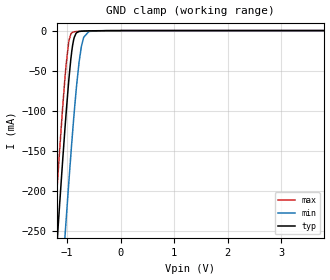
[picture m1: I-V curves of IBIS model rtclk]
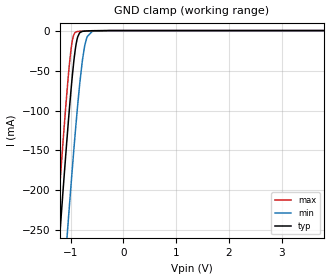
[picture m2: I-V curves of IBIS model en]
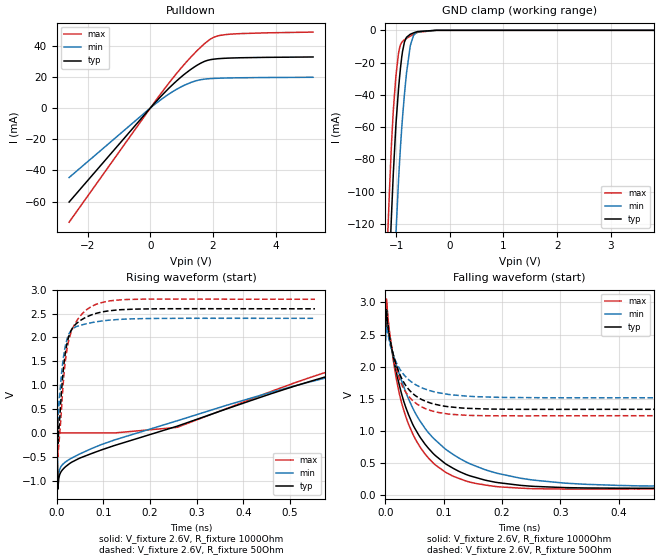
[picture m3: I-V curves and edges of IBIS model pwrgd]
|Texas Instruments Incorporated
| automotive Catalog 2.95V to 6V Input, 4A, 2MHz Synchronous Step Down
| SWIFT(tm) DCDC Converter
| Marketing part#   Digital Voltage Range   Package-type   #pins
| TPS57114QRTERQ1   2.95V-6V   QFN   16
[IBIS Ver]   4.1
[File name]   tps57114.ibs
[File Rev]   1.1
[Date]   8/06/2014
[Source]
| Texas Instruments Incorporated.
| Analog-eLab Design Center, HPA
| 12500 TI Blvd
| Dallas, TX -75243
[Notes]   Revision History:
| Rev 1.1: 8/06/2014
| - Added en, pwrgd models.
| Rev 1.0: 7/30/2014
| - Initial version of the model
| - Model generated from simulations in TISPICE
| - Model matched to SPICE simulation
| - C_comp although listed in numerical order of value are
|   obtained from varying PVT conditions. For PVT conditions for
|   each specific value refer the buffer description under
|   respective [Model]. IBIS model user is responsible for using
|   appropriate C_comp to simulate for Signal Integrity.
[Disclaimer]
| This model is designed as an aid for customers of Texas Instruments.
| TI and its licensors and suppliers make no warranties, either expressed
| or implied, with respect to this  model, including the warranties of
| merchantability or fitness for a particular purpose. The model is
| provided solely on an "as is" basis. The entire risk as to its quality
| and performance is with the customer.
[Copyright]
(C) Copyright 2014 Texas Instruments Incorporated.All rights reserved.
|   TPS57114
[Component]   TPS57114RTE
[Manufacturer]   TI
[Package]   |16 QFN  -  RTE package
|   typ   min   max
R_pkg   0.02609   0.02582   0.02655
L_pkg   0.81078nH   0.79906nH   0.82662nH
C_pkg   0.15670pF   0.14661pF   0.16188pF
[Pin]  signal_name   model_name   R_pin   L_pin   C_pin
1   VIN   power   0.01187   0.75296nH  0.26060pF
2   VIN   power   0.01171   0.71361nH  0.26727pF
3   GND   gnd   0.01169   0.71205nH  0.26671pF
4   GND   gnd   0.01220   0.73983nH  0.28477pF
5   GND   gnd   0.03032   0.96192nH  0.16334pF
6   VSENSE   nc   0.02662   0.83091nH  0.16437pF
7   COMP   nc   0.02547   0.78920nH  0.15897pF
8   RT/CLK   rtclk   0.02655   0.82662nH  0.14661pF
9   SS/TR   nc   0.02579   0.79643nH  0.14300pF
10   PH   nc   0.01088   0.65997nH  0.25329pF
11   PH   nc   0.01090   0.63864nH  0.27183pF
12   PH   nc   0.01125   0.71480nH  0.24611pF
13   BOOT   nc   0.02895   0.90385nH  0.15593pF
14   PWRGD   pwrgd   0.02582   0.79906nH  0.16162pF
15   EN   en   0.02591   0.80666nH  0.16188pF
16   VIN   power   0.02908   0.91969nH  0.15877pF
| Models and submodels in the file (3): rtclk (Input), en (Input), pwrgd (Open_drain)
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|   rtclk Model
[Model]   rtclk
Model_type   Input
Vinl = 0.4
Vinh = 2.5
|   typ   min   max
|   (nom PVT)   (fast PVT)   (slow PVT)
C_comp   1.701e-13   1.679e-13   1.709e-13
| Where nom  PVT is Nominal Process, 2.6V, 27C
|   Fast PVT is Strong Process,  2.8V, -40C
|   Slow PVT is Weak Process,   2.4V, 150C
[Voltage Range]   2.6   2.4   2.8
|Junction Temperature
[Temperature Range]   27   150   -40
[Power Clamp Reference]   2.6   2.4   2.8
[GND Clamp Reference]   0   0   0
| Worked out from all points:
|   GND clamp passes 1 mA (typ) near -0.77 V on its own axis
[GND Clamp]
|   Voltage   I(typ)   I(min)   I(max)
-2.6V     -1.785A    -1.914A    -1.724A
-1.269V   -345mA     -484.1mA   -276.9mA
-1.232V   -307.3mA   -446.4mA   -239.1mA
-1.169V   -243.8mA   -382.6mA   -175.9mA
-1.045V   -124.9mA   -260mA     -61.44mA
-1.024V   -105.6mA   -239.3mA   -44.69mA
-972.8mV  -63.71mA   -191.7mA   -14.71mA
-898.4mV  -18.16mA   -125.9mA   -2.023mA
-826.4mV  -2.757mA   -69.8mA    -1.176mA
-735.2mV  -741uA     -19.94mA   -820.7uA
-593.6mV  -320.7uA   -1.006mA   -410.6uA
5.2V      0A         0A         0A
[POWER Clamp]
|   Voltage   I(typ)   I(min)   I(max)
-2.6V     0A         0A         0A
0V        0A         0A         0A
5.2V      0A         0A         0A
|   en Model
[Model]   en
Model_type   Input
Vinl = 0.4
Vinh = 2.5
|   typ   min   max
|   (nom PVT)   (fast PVT)   (slow PVT)
C_comp   1.654e-13   1.644e-13   1.679e-13
| Where nom  PVT is Nominal Process, 2.6V, 27C
|   Fast PVT is Strong Process,  2.8V, -40C
|   Slow PVT is Weak Process,   2.4V, 150C
[Voltage Range]   2.6   2.4   2.8
|Junction Temperature
[Temperature Range]   27   150   -40
[Power Clamp Reference]   2.6   2.4   2.8
[GND Clamp Reference]   0   0   0
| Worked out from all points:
|   GND clamp passes 1 mA (typ) near -0.78 V on its own axis
[GND Clamp]
|   Voltage   I(typ)   I(min)   I(max)
-2.6V     -1.608A    -1.726A    -1.554A
-1.266V   -310.5mA   -436.6mA   -248.7mA
-1.232V   -278.9mA   -405.1mA   -217.1mA
-1.172V   -224.3mA   -350.2mA   -162.6mA
-1.085V   -148mA     -272.3mA   -87.92mA
-1.043V   -112.4mA   -235mA     -54.82mA
-970.4mV  -57.53mA   -173.6mA   -12.98mA
-897mV    -16.81mA   -115.1mA   -1.668mA
-824mV    -2.466mA   -63.66mA   -865uA
-732.8mV  -615.5uA   -18.38mA   -530.6uA
-591.2mV  -215.8uA   -921.1uA   -150.8uA
5.2V      0A         0A         0A
[POWER Clamp]
|   Voltage   I(typ)   I(min)   I(max)
-2.6V     0A         0A         0A
0V        0A         0A         0A
5.2V      0A         0A         0A
|   pwrgd Model
[Model]   pwrgd
Model_type   Open_drain
Polarity   Inverting
Vmeas = 1.3
Vref = 2.6
Cref = 2pF
Rref = 100
|   typ   min   max
|   (nom PVT)   (fast PVT)   (slow PVT)
C_comp   3.259e-13   2.888e-13   3.619e-13
| Where nom  PVT is Nominal Process, 2.6V, 27C
|   Fast PVT is Strong Process,  2.8V, -40C
|   Slow PVT is Weak Process,   2.4V, 150C
[Voltage Range]   2.6   2.4   2.8
|Junction Temperature
[Temperature Range]   27   125   -40
[Pullup Reference]   2.6   2.4   2.8
[Pulldown Reference]   0   0   0
[Power Clamp Reference]   2.6   2.4   2.8
[GND Clamp Reference]   0   0   0
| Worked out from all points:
|   slope of the pulldown table from 0 to 0.39 V, typ, clamps not added: 45.7 ohm
|   GND clamp passes 1 mA (typ) near -0.62 V on its own axis
|   falling waveform, V_fixture 2.6V, R_fixture 1000Ohm: 20-80 % time 71.7ps typ, 102ps min, 56.8ps max; typ from 2.6 V to 0.11 V
|   rising waveform, V_fixture 2.6V, R_fixture 1000Ohm: 20-80 % time 651ps typ, 685ps min, 624ps max; typ from 0.11 V to 2.6 V
|   falling waveform, V_fixture 2.6V, R_fixture 50Ohm: 20-80 % time 36.6ps typ, 45.5ps min, 31.3ps max; typ from 2.6 V to 1.33 V
|   rising waveform, V_fixture 2.6V, R_fixture 50Ohm: 20-80 % time 32.4ps typ, 25.3ps min, 34.7ps max; typ from 1.33 V to 2.6 V
[Pulldown]
|   Voltage   I(typ)   I(min)   I(max)
-2.6V     -60.31mA   -44.62mA   -73.23mA
0V        0A         0A         0A
362.4mV   7.97mA     5.688mA    9.925mA
755.2mV   15.79mA    10.96mA    20.06mA
1.11V     21.95mA    14.76mA    28.54mA
1.51V     27.57mA    17.67mA    37.06mA
1.832V    30.51mA    18.65mA    42.83mA
2.121V    31.46mA    18.99mA    45.96mA
2.546V    31.96mA    19.22mA    47.25mA
5.2V      32.64mA    19.64mA    48.59mA
[GND Clamp]
|   Voltage   I(typ)   I(min)   I(max)
-2.6V     -1.679A    -1.742A    -1.651A
-1.15V    -168.7mA   -250.5mA   -120.9mA
-1.091V   -118mA     -197.7mA   -73.51mA
-1.052V   -88.15mA   -164.2mA   -49.32mA
-1.001V   -57.14mA   -124.5mA   -27.39mA
-941.6mV  -31.06mA   -84.74mA   -11.68mA
-881.4mV  -13.22mA   -54.21mA   -6.899mA
-807.2mV  -4.322mA   -26.62mA   -4.999mA
-735.8mV  -2.419mA   -9.464mA   -3.555mA
-624.8mV  -1.007mA   -1.336mA   -1.624mA
-260mV    -246.8nA   -3.093uA   -51.13nA
5.2V      0A         0A         0A
[POWER Clamp]
|   Voltage   I(typ)   I(min)   I(max)
-2.6V     0A         0A         0A
0V        0A         0A         0A
5.2V      0A         0A         0A
[Ramp]
R_load = 1000
|   typ   min   max
dV/dt_r   1.49325/6.49618e-10   1.35616/6.82854e-10   1.62132/6.2478e-10
dV/dt_f   1.4939/7.16963e-11   1.35674/1.01541e-10   1.6218/5.68186e-11
[Falling Waveform]
V_fixture = 2.6V
V_fixture_min = 2.4V
V_fixture_max = 2.8V
R_fixture = 1000Ohm
|   Time   V(typ)   V(min)   V(max)
0s        2.6V       2.4V       2.8V
2ps       2.899V     2.732V     3.053V
8ps       2.429V     2.387V     2.468V
20ps      1.863V     1.989V     1.749V
34ps      1.388V     1.624V     1.248V
50ps      1.044V     1.297V     893.4mV
86ps      610mV      852.4mV    464.2mV
146ps     293.5mV    480.5mV    196mV
344ps     107.3mV    164.4mV    88.81mV
1.096ns   110.3mV    138.2mV    97.27mV
[Rising Waveform]
V_fixture = 2.6V
V_fixture_min = 2.4V
V_fixture_max = 2.8V
R_fixture = 1000Ohm
|   Time   V(typ)   V(min)   V(max)
0s        110.1mV    138.7mV    96.97mV
2ps       -1.178V    -1.054V    0V
8ps       -827.8mV   -716.7mV   0V
32ps      -611.5mV   -524.6mV   0V
258ps     140.6mV    254.1mV    117mV
624ps     1.305V     1.26V      1.413V
914ps     1.918V     1.781V     2.093V
1.32ns    2.349V     2.16V      2.553V
2.042ns   2.56V      2.358V     2.763V
3.998ns   2.599V     2.399V     2.799V
[Falling Waveform]
V_fixture = 2.6V
V_fixture_min = 2.4V
V_fixture_max = 2.8V
R_fixture = 50Ohm
|   Time   V(typ)   V(min)   V(max)
0s        2.6V       2.4V       2.8V
2ps       2.861V     2.692V     3.02V
6ps       2.519V     2.427V     2.605V
12ps      2.241V     2.216V     2.248V
20ps      1.989V     2.039V     1.925V
30ps      1.779V     1.893V     1.68V
50ps      1.557V     1.728V     1.445V
78ps      1.43V      1.621V     1.314V
190ps     1.337V     1.522V     1.232V
554ps     1.335V     1.515V     1.235V
[Rising Waveform]
V_fixture = 2.6V
V_fixture_min = 2.4V
V_fixture_max = 2.8V
R_fixture = 50Ohm
|   Time   V(typ)   V(min)   V(max)
0s        1.335V     1.515V     1.234V
2ps       -222.7mV   189.7mV    -495.8mV
8ps       594.9mV    1.031V     229.2mV
12ps      1.133V     1.432V     827.4mV
18ps      1.67V      1.82V      1.497V
24ps      1.97V      2.033V     1.877V
42ps      2.293V     2.228V     2.34V
72ps      2.465V     2.305V     2.635V
150ps     2.586V     2.386V     2.795V
554ps     2.6V       2.4V       2.8V
